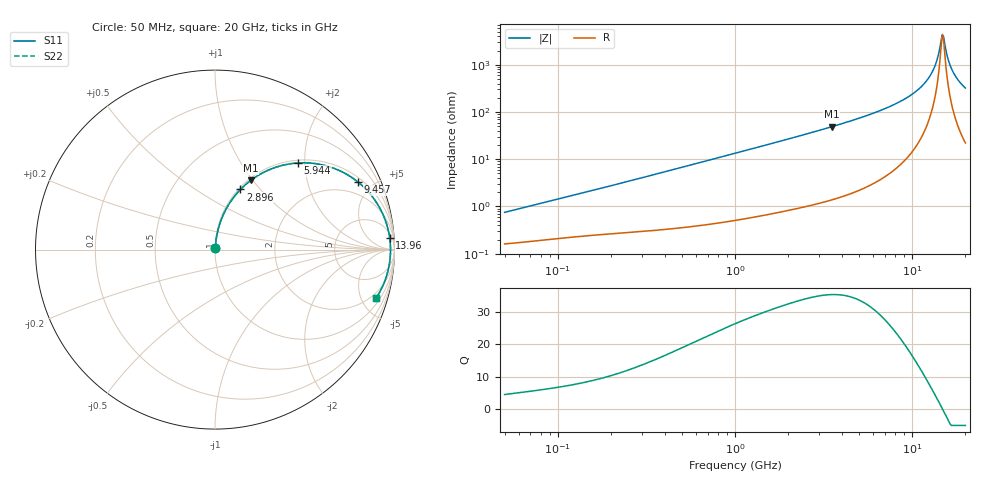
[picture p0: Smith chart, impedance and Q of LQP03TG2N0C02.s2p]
!Murata Part Number: LQP03TG2N0C02
!These Parameters are Measured in Series Mode Connection
!  o--[Z]--o
!Port1  Port2
!  o-------o
!Freq. Start=50[MHz] Stop=20[GHz], 401[Steps]
# Hz S RI R 50
!Freq.(Hz) S11(Real) S11(Imag) S21(Real) S21(Imag) S12(Real) S12(Imag) S22(Real) S22(Imag)
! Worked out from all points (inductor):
!   401 points, 50 MHz to 20 GHz, reference 50 ohm
!   read as one part in series: L = 2.31 nH near 51.52 MHz
!   highest Q = 35.4 at 3.519 GHz (marker M1), where L = 2.21 nH
!   self-resonance near 14.82 GHz
!   S11 on the Smith chart (normalised r, x): 50 MHz: 1.00, +0.01; 2.896 GHz: 1.02, +0.79; 5.944 GHz: 1.06, +1.85; 9.457 GHz: 1.22, +4.13; 13.96 GHz: 10, +27; 20 GHz: 1.44, -6.43
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5e7  0.00166 0.00731  0.9983 -0.00731  0.9983 -0.00731  0.00166 0.00731
1.364002e8  0.0027 0.019  0.9973 -0.019  0.9973 -0.019  0.0027 0.019
3.721004e8  0.00567 0.0499  0.9943 -0.0499  0.9943 -0.0499  0.00567 0.0499
1e9  0.0223 0.13  0.9777 -0.13  0.9777 -0.13  0.0223 0.13
2.728004e9  0.1278 0.3197  0.8722 -0.3197  0.8722 -0.3197  0.1278 0.3197
2.896447e9  0.142 0.335  0.858 -0.335  0.858 -0.335  0.142 0.335
3.519108e9  0.1992 0.3855  0.8008 -0.3855  0.8008 -0.3855  0.1992 0.3855
5.944466e9  0.4613 0.4828  0.5387 -0.4828  0.5387 -0.4828  0.4613 0.4828
7.442007e9  0.6216 0.4662  0.3784 -0.4662  0.3784 -0.4662  0.6216 0.4662
9.457416e9  0.7977 0.3757  0.2023 -0.3757  0.2023 -0.3757  0.7977 0.3757
1.098561e10  0.8905 0.2761  0.1095 -0.2761  0.1095 -0.2761  0.8905 0.2761
1.220001e10  0.9389 0.189  0.0611 -0.189  0.0611 -0.189  0.9389 0.189
1.314879e10  0.9624 0.1202  0.0376 -0.1202  0.0376 -0.1202  0.9624 0.1202
1.396067e10  0.9737 0.0625  0.0263 -0.0625  0.0263 -0.0625  0.9737 0.0625
1.460232e10  0.9776 0.0184  0.0224 -0.0184  0.0224 -0.0184  0.9776 0.0184
1.482269e10  0.978 0.00368  0.022 -0.00368  0.022 -0.00368  0.978 0.00368
1.504638e10  0.9779 -0.0111  0.0221 0.0111  0.0221 0.0111  0.9779 -0.0111
1.527346e10  0.9775 -0.0259  0.0225 0.0259  0.0225 0.0259  0.9775 -0.0259
1.621653e10  0.971 -0.0845  0.029 0.0845  0.029 0.0845  0.971 -0.0845
1.696185e10  0.9616 -0.1276  0.0384 0.1276  0.0384 0.1276  0.9616 -0.1276
1.828096e10  0.9377 -0.1964  0.0623 0.1964  0.0623 0.1964  0.9377 -0.1964
2e10  0.8966 -0.2719  0.1034 0.2719  0.1034 0.2719  0.8966 -0.2719
